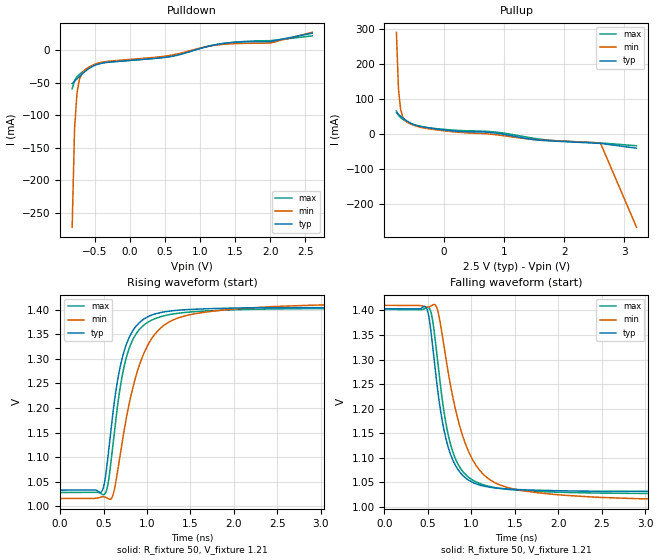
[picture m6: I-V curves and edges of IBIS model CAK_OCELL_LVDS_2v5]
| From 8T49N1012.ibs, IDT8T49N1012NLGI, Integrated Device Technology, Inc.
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[Model] CAK_OCELL_LVDS_2v5
Model_type   Output
Polarity   Non-Inverting
|   typ   min   max
C_comp   2pF   1.5pF   2.5pF
Vmeas = 1.218V
Rref = 50
Cref = 0
Vref = 1.218V
|   typ   min   max
[Voltage range]   2.5V   2.375V   2.625V
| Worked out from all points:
|   slope of the pulldown table from 0 to 0.375 V, typ, clamps not added: 113 ohm
|   slope of the pullup table from 0 to 0.375 V, typ, clamps not added: 78.1 ohm
|   rising waveform, R_fixture 50, V_fixture 1.21: 20-80 % time 208ps typ, 338ps min, 214ps max; typ from 1.03 V to 1.4 V
|   falling waveform, R_fixture 50, V_fixture 1.21: 20-80 % time 208ps typ, 338ps min, 214ps max; typ from 1.4 V to 1.03 V
[Pulldown]
|Voltage   I (typ)   I (min)   I (max)
|Note, modeling breaks down at 250mA and above.  This is well beyond the functional   |
|operating range of the device.  Should this scenario occur, catastrophic failure and   |
|possible damage to the device and/or board is of higher concern than the I-V curve   |
|behavior.  The IBIS checker will flag currents in excess of 10A with warnings.  Lines   |
|with currents in excess of 0.35 A have been commented out.  The points still remain|
|available to the user if the user desires to use them.   |
|-2.20000e+00   -1.76153e+01   -1.29939e+01   -1.46994e+01
|-1.90000e+00   -1.33479e+01   -1.02078e+01   -1.13564e+01
|-1.60000e+00   -9.08003e+00   -7.42145e+00   -8.01343e+00
|-1.30000e+00   -4.81016e+00   -4.63709e+00   -4.67118e+00
|-1.00000e+00   -5.46982e-01   -1.85388e+00   -1.32964e+00
|-9.99000e-01   -5.32790e-01   -1.84461e+00   -1.31851e+00
|-9.64529e-01   -1.72445e-01   -1.52489e+00   -9.34973e-01
|-9.30057e-01   -8.24515e-02   -1.20522e+00   -5.51611e-01
|-8.95586e-01   -6.19842e-02   -8.85622e-01   -2.22624e-01
|-8.61115e-01   -5.52796e-02   -5.66114e-01   -9.67861e-02
-826.6mV  -51.28mA   -271.7mA   -59.31mA
-792.2mV  -47.73mA   -120.4mA   -46.7mA
-757.7mV  -44.12mA   -65.85mA   -41mA
-723.2mV  -40.5mA    -45mA      -37.24mA
-688.8mV  -37.01mA   -36.03mA   -34.13mA
-619.8mV  -30.76mA   -28.24mA   -28.79mA
-516.4mV  -23.95mA   -22.18mA   -22.78mA
-378.5mV  -19.53mA   -18.01mA   -19.03mA
586.7mV   -9.754mA   -7.688mA   -9.042mA
1.311V    10.09mA    8.752mA    9.876mA
2.001V    13.25mA    11mA       14.57mA
2.601V    26.12mA    27.42mA    21.91mA
| 3.20060e+00   5.76461e-02   6.52581e-01   4.63281e-02
| 3.80040e+00   8.46015e+00   1.01451e+01   5.83527e+00
| 4.40020e+00   2.30830e+01   1.96842e+01   1.72767e+01
| 5.00000e+00   3.77286e+01   2.92374e+01   2.87380e+01
[Pullup]
|Voltage   I (typ)   I (min)   I (max)
|Note, modeling breaks down at 250mA and above.  This is well beyond the functional   |
|operating range of the device.  Should this scenario occur, catastrophic failure and   |
|possible damage to the device and/or board is of higher concern than the I-V curve   |
|behavior.  The IBIS checker will flag currents in excess of 10A with warnings.  Lines   |
|with currents in excess of 0.35 A have been commented out.  The points still remain|
|available to the user if the user desires to use them.   |
|-2.20000e+00   3.04159e+01   2.24791e+01   2.54060e+01
|-1.90000e+00   2.30868e+01   1.76998e+01   1.96688e+01
|-1.60000e+00   1.57638e+01   1.29235e+01   1.39348e+01
|-1.30000e+00   8.45063e+00   8.15131e+00   8.20765e+00
|-1.00000e+00   1.14106e+00   3.38593e+00   2.48764e+00
|-9.99000e-01   1.11670e+00   3.37005e+00   2.46858e+00
|-9.64529e-01   4.05964e-01   2.82287e+00   1.81163e+00
|-9.30057e-01   1.40036e-01   2.27574e+00   1.15474e+00
|-8.95586e-01   8.58073e-02   1.72865e+00   5.49652e-01
|-8.61115e-01   7.21896e-02   1.18159e+00   2.05254e-01
|-8.26644e-01   6.61669e-02   6.57712e-01   9.77218e-02
-792.2mV  61.36mA    290.1mA    65.67mA
-757.7mV  56.4mA     128.5mA    53.75mA
-723.2mV  51.31mA    71.28mA    47.24mA
-688.8mV  46.43mA    49.57mA    42.52mA
-619.8mV  37.81mA    34.89mA    35.42mA
-516.4mV  28.22mA    26.16mA    27.8mA
-413mV    23.02mA    20.57mA    22.72mA
69.61mV   10.56mA    8.161mA    12.57mA
793.5mV   4.472mA    -351uA     6.925mA
1.586V    -17.28mA   -16.33mA   -14.12mA
2.601V    -26.35mA   -25.19mA   -25.05mA
3.201V    -40mA      -265mA     -33.02mA
| 3.80040e+00   -4.79871e+00   -5.78252e+00   -3.27035e+00
| 4.40020e+00   -1.33176e+01   -1.13428e+01   -9.93824e+00
| 5.00000e+00   -2.18424e+01   -1.69072e+01   -1.66137e+01
[Ramp]
|   typ   min   max
dV/dt_r   0.225/0.209n   0.237/0.338n   0.227/0.214n
dV/dt_f   0.225/0.209n   0.237/0.338n   0.227/0.214n
R_load =   50.0000
[Rising Waveform]
R_fixture = 50
V_fixture = 1.21   |Vcc_typ
V_fixture_min = 1.199 |Vcc_min
V_fixture_max = 1.21 |Vcc_max
C_fixture = 0.0p
| Time   typ   min   max
0s        1.033V     1.016V     1.028V
480ps     1.03V      1.019V     1.024V
537.8ps   1.082V     1.017V     1.035V
595.6ps   1.173V     1.017V     1.106V
680ps     1.274V     1.092V     1.229V
760ps     1.328V     1.178V     1.301V
1.004ns   1.385V     1.326V     1.374V
1.231ns   1.396V     1.372V     1.389V
1.604ns   1.401V     1.393V     1.397V
4ns       1.403V     1.41V      1.402V
[Falling Waveform]
R_fixture = 50
V_fixture = 1.21   |Vcc_typ
V_fixture_min = 1.199 |Vcc_min
V_fixture_max = 1.21 |Vcc_max
C_fixture = 0.0p
| Time   typ   min   max
0s        1.403V     1.41V      1.402V
480ps     1.406V     1.407V     1.406V
537.8ps   1.355V     1.409V     1.395V
595.6ps   1.263V     1.409V     1.323V
680ps     1.162V     1.334V     1.201V
760ps     1.108V     1.248V     1.128V
1ns       1.051V     1.101V     1.057V
1.227ns   1.04V      1.054V     1.041V
1.596ns   1.035V     1.033V     1.033V
4ns       1.033V     1.016V     1.028V
